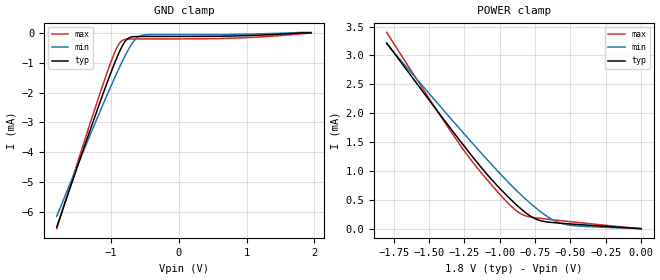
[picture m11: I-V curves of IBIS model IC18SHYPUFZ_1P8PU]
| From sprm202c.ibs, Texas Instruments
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|   Model IC18SHYPUFZ_1P8PU
[Model]   IC18SHYPUFZ_1P8PU
Model_type   Input
Polarity   Non-Inverting
Vinl =   0.8400V
Vinh =   0.9800V
C_comp   0.8000pF   0.9300pF   0.6600pF
[Model Spec]
|   typ   min   max
Vinh   0.98V   0.86V   1.05V
Vinl   0.84V   0.70V   0.91V
[Temperature Range]   25.0000   0.1250k   -40.0000
[Voltage Range]   1.8000V   1.6200V   1.9500V
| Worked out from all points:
|   GND clamp passes 1 mA (typ) near -0.94 V on its own axis
|   POWER clamp passes 1 mA (typ) near -1.11 V on its own axis
[GND_clamp]
| voltage   I(typ)   I(min)   I(max)
-1.8V     -6.507mA   -6.146mA   -6.559mA
-1.4V     -3.858mA   -3.927mA   -3.681mA
-1.08V    -1.809mA   -2.199mA   -1.478mA
-920mV    -864.7uA   -1.375mA   -522.9uA
-880mV    -653.6uA   -1.178mA   -357.3uA
-840mV    -463.9uA   -985.7uA   -260.2uA
-760mV    -203.2uA   -626.2uA   -209uA
-680mV    -129.6uA   -324.4uA   -203.5uA
-600mV    -121.1uA   -133.2uA   -202.9uA
-520mV    -120.2uA   -68.08uA   -202.6uA
840mV     -100.6uA   -46.43uA   -172.2uA
1.95V     250pA      17.25uA    0A
[POWER_clamp]
| voltage   I(typ)   I(min)   I(max)
-1.8V     3.216mA    3.2mA      3.399mA
-1.44V    2.032mA    2.17mA     2.03mA
-1.24V    1.392mA    1.609mA    1.309mA
-1.12V    1.027mA    1.279mA    936.1uA
-1.02V    750.4uA    1.011mA    650.2uA
-880mV    408.2uA    657.4uA    305.7uA
-820mV    282.1uA    518.8uA    224.3uA
-740mV    161.6uA    349.5uA    186.4uA
-640mV    109.4uA    174.5uA    158.2uA
-560mV    92.71uA    87.71uA    136.7uA
-440mV    71.22uA    44.74uA    105.5uA
0V        235.1pA    208.3pA    268.3pA
